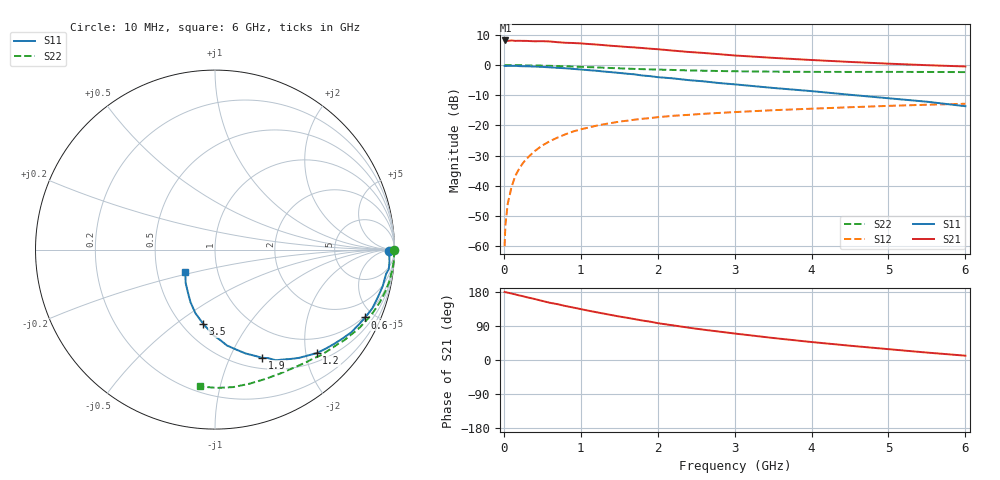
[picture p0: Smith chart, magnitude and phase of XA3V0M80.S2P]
! SIEMENS Discrete & RF Semiconductors
! BFY180
! Si NPN RF Bipolar Junction Transistor in MICRO-X
! VCE = 3 V  IC = 0.8 mA
! Common Emitter S-Parameters:  May  1997
# GHz  S  MA  R  50
!  f  S11  S21  S12  S22
! GHz  MAG  ANG  MAG  ANG  MAG  ANG  MAG  ANG
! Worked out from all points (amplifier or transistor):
!   36 points, 10 MHz to 6 GHz, reference 50 ohm
!   highest |S21| = 8.2 dB at 20 MHz (marker M1)
!   |S21| within 3 dB of that: start of sweep to 2.041 GHz
!   unconditionally stable (mu >= 1): 4.251 GHz to end of sweep
!   at 250 MHz: K = 0.08, MSG = 20.2 dB, |S12| = -32.4 dB
!   at 1.4 GHz: K = 0.47, MSG = 12.8 dB, |S12| = -19.2 dB
!   at 6 GHz: K = 1.05, MAG = 4.8 dB, |S12| = -12.8 dB
!   S11 on the Smith chart (normalised r, x): 10 MHz: 62, -10; 600 MHz: 0.92, -4.46; 1.2 GHz: 0.67, -2.22; 1.9 GHz: 0.63, -1.33; 3.5 GHz: 0.63, -0.63; 6 GHz: 0.70, -0.18
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0.01  0.9692 -0.3  2.546 179.7  0.001 87.1  0.9988 -0.2
0.02  0.9689 -1.0  2.564 178.9  0.0022 95.4  0.9999 -0.6
0.05  0.9718 -1.9  2.524 177.8  0.005 84.5  0.999 -1.3
0.1  0.974 -4.1  2.564 175.4  0.0096 87.3  0.9974 -2.6
0.15  0.9747 -6.4  2.525 173.1  0.0147 85.6  0.9981 -3.8
0.3  0.9568 -12.2  2.519 165.6  0.0285 81.1  0.9915 -7.6
0.5  0.9354 -20.5  2.496 155.9  0.0467 75.3  0.9816 -12.5
0.6  0.9186 -24.3  2.465 150.9  0.0551 72.9  0.9733 -14.9
0.9  0.8662 -34.9  2.327 138.5  0.0794 64.4  0.9478 -21.7
1.1  0.8258 -42.2  2.24 130.2  0.0922 59.2  0.9266 -25.9
1.2  0.8086 -45.5  2.196 126.2  0.099 57.2  0.9169 -28.1
1.5  0.7431 -55.0  2.048 114.8  0.1157 50.8  0.886 -33.7
1.9  0.6575 -66.5  1.874 101.2  0.1326 44.3  0.8506 -40.5
2  0.6323 -69.4  1.835 97.2  0.1371 42.8  0.8439 -42.0
2.2  0.6032 -73.6  1.74 91.4  0.1447 39.7  0.8321 -45.2
2.6  0.5383 -82.9  1.59 79.9  0.1562 35.0  0.8081 -50.8
2.8  0.5047 -86.7  1.517 74.9  0.1615 32.9  0.7989 -53.5
3.5  0.419 -99.0  1.32 58.1  0.1791 26.2  0.7798 -62.5
4  0.3709 -107.1  1.216 47.4  0.1897 21.9  0.7732 -68.9
4.5  0.3226 -115.1  1.13 37.7  0.2006 17.9  0.7715 -75.5
5.5  0.2476 -131.3  0.998 19.6  0.2207 9.8  0.7709 -89.3
6  0.2086 -142.5  0.95 11.4  0.2292 5.7  0.7665 -96.3
